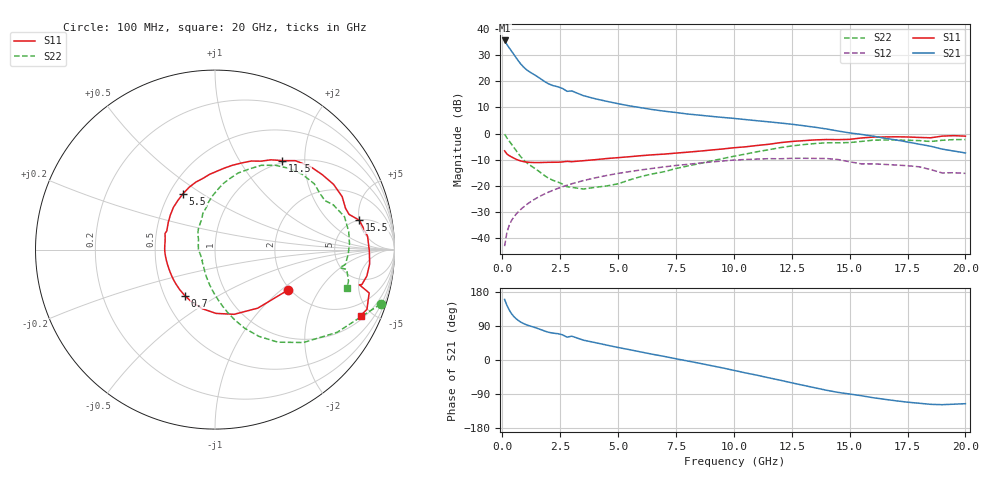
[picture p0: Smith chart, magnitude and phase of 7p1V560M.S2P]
! Infineon Technologies  Discrete & RF Semiconductors
! bfp620
! VCE =  1.5 V,  IC =  60 mA
! Common Emitter S-Parameters:  Sep 2002
# GHz  S  MA  R  50
!  f  S11  S21  S12  S22
! GHz  MAG  ANG  MAG  ANG  MAG  ANG  MAG  ANG
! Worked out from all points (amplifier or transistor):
!   59 points, 100 MHz to 20 GHz, reference 50 ohm
!   highest |S21| = 35.7 dB at 100 MHz (marker M1)
!   |S21| within 3 dB of that: start of sweep to 311.3 MHz
!   unconditionally stable (mu >= 1): 2.642 GHz to 2.958 GHz; 3.096 GHz to 9.881 GHz; 17.17 GHz to end of sweep
!   at 1 GHz: K = 0.87, MSG = 26.2 dB, |S12| = -27.6 dB
!   at 5.5 GHz: K = 1.04, MAG = 11.4 dB, |S12| = -14.6 dB
!   at 20 GHz: K = 1.30, MAG = 0.6 dB, |S12| = -15.3 dB
!   S11 on the Smith chart (normalised r, x): 100 MHz: 1.95, -1.12; 700 MHz: 0.63, -0.36; 5.5 GHz: 0.59, +0.42; 11.5 GHz: 0.96, +1.55; 15.5 GHz: 5.01, +5.03; 20 GHz: 1.21, -4.30
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0.1  0.4649 -29.0  60.98 159.9  0.0069 80.6  0.9718 -18.2
0.2  0.4041 -53.8  50.94 144.1  0.0127 72.7  0.8219 -34.1
0.3  0.376 -73.5  43.88 131.7  0.0174 69.4  0.7149 -46.4
0.4  0.3555 -89.1  38.01 122.1  0.0215 67.5  0.6236 -55.8
0.5  0.3368 -102.2  32.82 114.7  0.0251 66.2  0.5413 -63.2
0.6  0.3203 -113.4  28.31 108.8  0.0285 65.4  0.4687 -69.3
0.7  0.307 -123.2  24.54 103.9  0.0318 64.9  0.4072 -74.3
0.9  0.2902 -138.5  19.19 96.7  0.0383 64.2  0.3186 -82.3
1.1  0.282 -149.2  16.09 91.7  0.045 63.6  0.2654 -88.2
1.5  0.2772 -164.5  12.47 83.8  0.0584 61.7  0.2003 -98.3
1.9  0.2798 -177.7  9.494 75.0  0.0718 59.1  0.1479 -110.7
2.8  0.2925 162.1  6.45 60.3  0.1019 51.7  0.0951 -139.9
3  0.288 158.9  6.555 62.9  0.1086 49.9  0.0927 -138.9
3.5  0.3009 150.0  5.328 52.4  0.125 45.1  0.0861 -158.9
5.5  0.3591 119.6  3.387 27.2  0.186 25.4  0.129 138.3
7  0.4029 99.4  2.682 9.4  0.2293 10.5  0.1856 113.3
10.5  0.5555 62.5  1.851 -34.0  0.3174 -29.5  0.4032 78.4
11.5  0.621 53.0  1.677 -46.9  0.3292 -41.9  0.4877 67.0
13.5  0.7541 28.8  1.32 -73.3  0.3326 -65.9  0.6419 40.8
15.5  0.8208 11.5  0.963 -94.2  0.2618 -88.1  0.7048 20.7
17  0.8654 -5.3  0.753 -107.7  0.2487 -97.6  0.75 2.4
20  0.8905 -24.4  0.424 -115.3  0.172 -107.5  0.7661 -16.0
